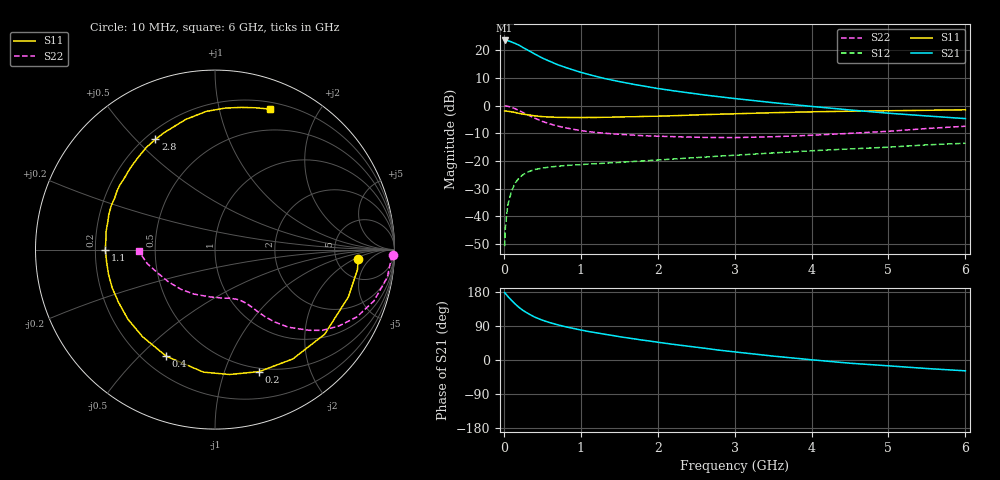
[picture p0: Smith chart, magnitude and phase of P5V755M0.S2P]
! SIEMENS Small Signal Semiconductors
! BFP183
! Si NPN RF Bipolar Junction Transistor in SOT143
! VCE = 0.75 V  IC = 5 mA
! Common Emitter S-Parameters:  March  1996
# GHz  S  MA  R  50
!  f  S11  S21  S12  S22
! GHz  MAG  ANG  MAG  ANG  MAG  ANG  MAG  ANG
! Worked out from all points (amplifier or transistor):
!   36 points, 10 MHz to 6 GHz, reference 50 ohm
!   highest |S21| = 23.5 dB at 10 MHz (marker M1)
!   |S21| within 3 dB of that: start of sweep to 278.7 MHz
!   unconditionally stable (mu >= 1): 1.432 GHz to end of sweep
!   at 250 MHz: K = 0.22, MSG = 22.9 dB, |S12| = -24.9 dB
!   at 1.4 GHz: K = 0.99, MSG = 14.9 dB, |S12| = -20.6 dB
!   at 6 GHz: K = 1.06, MAG = 2.9 dB, |S12| = -13.6 dB
!   S11 on the Smith chart (normalised r, x): 10 MHz: 8.23, -2.41; 200 MHz: 0.46, -1.32; 400 MHz: 0.29, -0.60; 1.1 GHz: 0.24, +0.00; 2.8 GHz: 0.24, +0.57; 6 GHz: 0.27, +1.43
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0.01  0.799 -3.8  14.97 178.0  0.0029 86.8  0.9899 -1.8
0.02  0.8017 -8.0  14.9 175.8  0.0063 84.6  0.9813 -3.7
0.05  0.7886 -19.5  14.85 168.3  0.0157 81.0  0.9724 -9.1
0.1  0.7718 -37.7  14.09 157.4  0.0288 69.8  0.9306 -17.9
0.15  0.7478 -54.6  13.18 147.2  0.0405 63.1  0.8748 -25.4
0.2  0.723 -70.1  12.26 138.3  0.0497 56.3  0.8106 -31.7
0.25  0.7005 -83.4  11.14 130.7  0.0566 50.3  0.7477 -37.0
0.3  0.6857 -95.4  10.21 124.5  0.0624 45.7  0.6895 -40.7
0.4  0.6529 -114.6  8.556 113.3  0.07 38.9  0.5939 -46.7
0.5  0.6313 -129.7  7.213 105.1  0.0745 34.3  0.519 -50.7
0.6  0.6212 -141.4  6.275 98.5  0.0778 31.4  0.4658 -53.3
0.7  0.6126 -151.2  5.468 92.9  0.0805 29.4  0.427 -55.1
0.9  0.609 -166.9  4.404 83.5  0.0848 27.2  0.3737 -57.8
1.1  0.6111 180.0  3.655 75.2  0.0882 26.0  0.3384 -60.6
1.5  0.6233 161.6  2.71 61.6  0.0942 25.8  0.3032 -66.0
1.8  0.636 149.2  2.27 52.6  0.1 26.2  0.2865 -71.3
2.2  0.6557 135.8  1.852 41.4  0.1084 26.1  0.2751 -79.6
2.8  0.6981 118.4  1.444 25.9  0.1224 25.6  0.265 -94.8
3.5  0.7434 102.6  1.128 10.3  0.1397 23.8  0.2737 -115.0
4.5  0.791 85.7  0.833 -8.5  0.1651 19.1  0.3151 -145.1
5.5  0.822 74.0  0.649 -22.5  0.1953 14.0  0.3854 -168.3
6  0.8398 68.8  0.582 -28.6  0.209 9.9  0.424 -178.7
